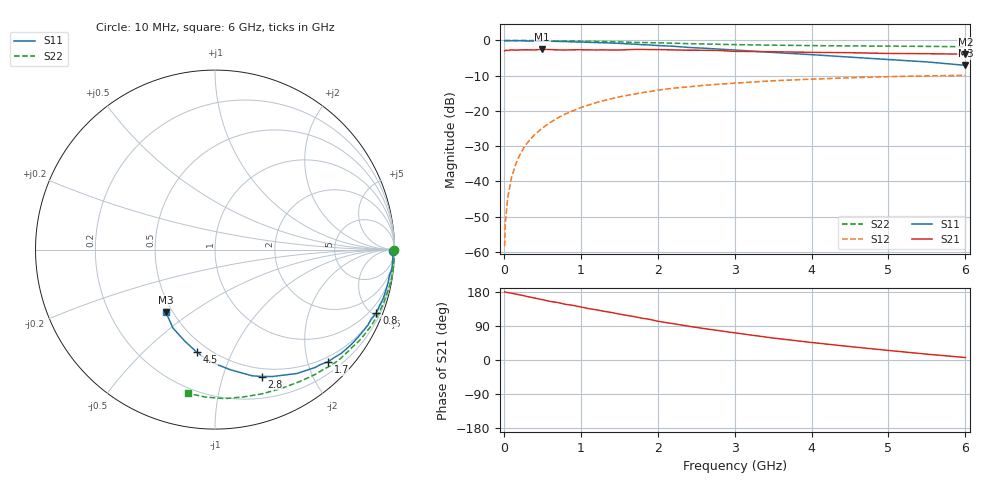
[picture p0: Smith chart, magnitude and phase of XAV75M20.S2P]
! SIEMENS Discrete & RF Semiconductors
! BFY180
! Si NPN RF Bipolar Junction Transistor in MICRO-X
! VCE = 0.75 V  IC = 0.2 mA
! Common Emitter S-Parameters:  May  1997
# GHz  S  MA  R  50
!  f  S11  S21  S12  S22
! GHz  MAG  ANG  MAG  ANG  MAG  ANG  MAG  ANG
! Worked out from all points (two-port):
!   36 points, 10 MHz to 6 GHz, reference 50 ohm
!   highest |S21| = -2.52 dB at 500 MHz (marker M1); lowest = -3.9 dB at 6 GHz (marker M2)
!   |S21| within 3 dB of the highest: start of sweep to end of sweep
!   lowest |S11| = -7.1 dB at 6 GHz (marker M3), VSWR 2.59, Z = 23 - j19.9 ohm
!   |S11| at or under -10 dB: nowhere
!   |S22| runs from -1.8 to 0.0 dB; largest |S21 - S12| = 0.74
!   S11 on the Smith chart (normalised r, x): 10 MHz: open; 800 MHz: 0.50, -5.25; 1.7 GHz: 0.40, -2.37; 2.8 GHz: 0.41, -1.35; 4.5 GHz: 0.43, -0.74; 6 GHz: 0.46, -0.40
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0.01  0.9897 -0.3  0.71 179.8  0.0012 84.0  0.9999 -0.2
0.02  0.9942 -0.6  0.725 179.1  0.0026 90.5  0.9999 -0.5
0.05  0.9909 -1.2  0.722 178.0  0.0058 87.1  0.9984 -1.1
0.1  0.9921 -2.6  0.735 176.3  0.0113 87.6  0.9988 -2.2
0.15  0.991 -4.2  0.728 174.2  0.017 85.9  0.9999 -3.2
0.2  0.9922 -5.4  0.733 172.0  0.0228 86.2  0.9977 -4.3
0.3  0.9825 -8.1  0.737 167.6  0.0346 82.7  0.9975 -6.4
0.4  0.9817 -10.8  0.733 163.5  0.0461 81.0  0.9971 -8.5
0.5  0.9786 -13.5  0.748 159.3  0.0569 78.5  0.9948 -10.7
0.8  0.9657 -21.4  0.732 147.1  0.0903 71.4  0.9855 -17.1
1.1  0.9406 -29.2  0.734 135.7  0.1209 64.2  0.9735 -23.4
1.4  0.9179 -37.0  0.731 125.3  0.1491 57.3  0.9574 -29.7
1.7  0.8871 -44.8  0.746 114.3  0.1732 50.9  0.9381 -35.4
2  0.8472 -52.2  0.742 102.3  0.1967 44.9  0.9258 -40.9
2.2  0.8277 -56.5  0.734 95.9  0.2099 40.9  0.9157 -44.6
2.4  0.7961 -61.5  0.727 89.3  0.2194 37.3  0.8997 -48.0
2.8  0.7534 -69.8  0.72 77.4  0.2396 30.7  0.8812 -54.4
3.5  0.6754 -82.6  0.691 58.0  0.2676 20.6  0.8573 -64.6
4  0.6286 -91.8  0.678 46.2  0.2825 13.6  0.8451 -71.9
4.5  0.5799 -100.2  0.67 35.4  0.2949 7.3  0.8362 -79.1
5.5  0.4958 -118.2  0.648 15.4  0.3139 -4.9  0.8234 -93.6
6  0.443 -128.3  0.639 6.5  0.3199 -11.1  0.8148 -100.8
